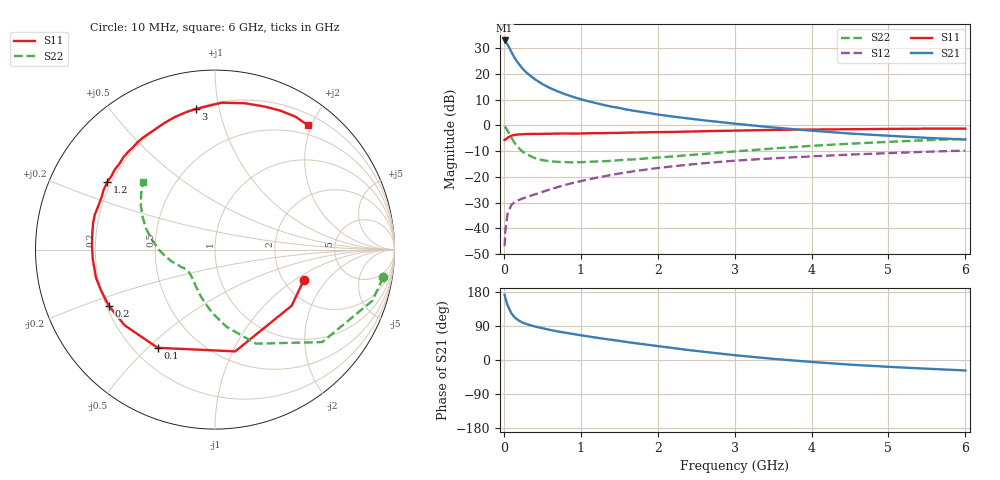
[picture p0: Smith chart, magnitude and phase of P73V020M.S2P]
! SIEMENS Small Signal Semiconductors
! BFP196
! Si NPN RF Bipolar Junction Transistor in SOT143
! VCE = 3 V  IC = 20 mA
! Common Emitter S-Parameters:  May  1996
# GHz  S  MA  R  50
!  f  S11  S21  S12  S22
! GHz  MAG  ANG  MAG  ANG  MAG  ANG  MAG  ANG
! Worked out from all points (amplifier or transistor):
!   36 points, 10 MHz to 6 GHz, reference 50 ohm
!   highest |S21| = 33.0 dB at 10 MHz (marker M1)
!   |S21| within 3 dB of that: start of sweep to 72.77 MHz
!   unconditionally stable (mu >= 1): 681.3 MHz to 3.325 GHz
!   at 250 MHz: K = 0.60, MSG = 25.1 dB, |S12| = -28.4 dB
!   at 1.4 GHz: K = 1.11, MAG = 11.2 dB, |S12| = -19.2 dB
!   at 6 GHz: K = 0.97, MSG = 2.1 dB, |S12| = -9.8 dB
!   S11 on the Smith chart (normalised r, x): 10 MHz: 2.56, -1.19; 100 MHz: 0.29, -0.54; 200 MHz: 0.21, -0.24; 1.2 GHz: 0.18, +0.28; 3 GHz: 0.20, +0.85; 6 GHz: 0.36, +1.95
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0.01  0.523 -18.9  44.82 172.3  0.0045 83.9  0.9499 -9.4
0.02  0.5295 -36.2  43 163.5  0.0091 74.0  0.9219 -18.0
0.05  0.5781 -78.8  37.01 143.6  0.0198 60.5  0.7889 -40.8
0.1  0.6336 -120.3  26.39 122.5  0.0288 45.9  0.5719 -66.4
0.15  0.6567 -140.0  19.44 110.8  0.0331 41.2  0.4364 -81.3
0.2  0.6696 -152.2  15.27 103.4  0.0358 40.4  0.3559 -92.1
0.25  0.6749 -160.7  12.37 98.1  0.0382 40.6  0.3035 -100.4
0.3  0.6815 -166.8  10.45 94.5  0.0407 42.2  0.2732 -106.7
0.4  0.6831 -175.5  7.965 88.7  0.0455 44.9  0.2323 -117.0
0.5  0.6856 178.2  6.378 83.9  0.0509 47.8  0.2115 -124.4
0.6  0.6892 172.9  5.333 79.5  0.0572 49.7  0.2007 -129.8
0.7  0.695 167.7  4.6 75.4  0.0633 51.3  0.1958 -134.2
0.8  0.6975 163.7  4.024 72.0  0.0698 51.7  0.1934 -137.8
1.1  0.704 151.8  2.946 62.2  0.0893 52.9  0.196 -145.3
1.2  0.7085 147.9  2.708 59.1  0.096 52.8  0.1987 -147.5
1.6  0.7241 134.9  2.031 47.4  0.1226 50.2  0.2156 -154.4
2.2  0.7468 117.5  1.484 31.6  0.1608 44.1  0.2498 -164.5
3  0.791 97.7  1.083 12.7  0.2063 34.3  0.3119 -179.8
3.5  0.8192 87.5  0.913 3.1  0.2294 28.1  0.3557 171.1
4.5  0.8436 70.9  0.696 -12.2  0.2711 16.8  0.4415 155.9
5.5  0.8659 58.7  0.573 -23.0  0.3079 5.9  0.5161 142.9
6  0.8647 53.1  0.533 -27.6  0.3249 0.0  0.5488 136.7
